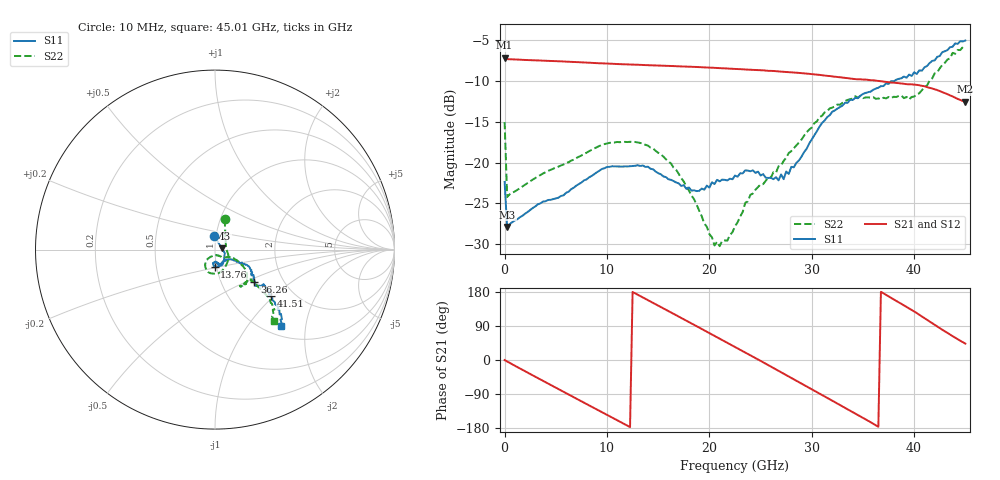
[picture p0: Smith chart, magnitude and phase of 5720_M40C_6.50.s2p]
! Device:  ADRF5720
! Description: 0.5dB LSB GaAs MMIC 6-bit Digital Attenuator
! Frequency:  0.000009 -  40 GHz
! Ports:
!	RF1	= Port 1
!	RF2	= Port 2
! Vdd:  3.3 Volt
! Vss:  -3.3 Volt
! Control:  0/3.3 Volt
! State:  6.50 dB attenuation
! Data:  The device was measured using G-S-G Probes on a matrix board.
!  Data was collected using an calibrated 4 port network analyzer.
!  The reference plane for this measurement is at the launchers.
! Note:  Analog Devices supplies this data as a sample of measured data
!  for this product.  Your particular data for this product may vary.
!  Data was taken at -40 degrees C.
!  Analog Devices reserves the right to change this data at anytime.
# GHZ S DB R 45.0
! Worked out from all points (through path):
!   181 points, 10 MHz to 45.01 GHz, reference 45 ohm
!   highest |S21| = -7.14 dB at 10 MHz (marker M1); lowest = -12.5 dB at 45.01 GHz (marker M2)
!   group delay of S21, straight-line fit = 41.3 ps
!   lowest |S11| = -27.9 dB at 260 MHz (marker M3), VSWR 1.08, Z = 48.7 + j0.608 ohm
!   |S11| at or under -10 dB: start of sweep to 38.04 GHz
!   |S22| runs from -30.2 to -5.8 dB; largest |S21 - S12| = 0.0017
!   S11 on the Smith chart (normalised r, x): 10 MHz: 0.98, +0.15; 13.76 GHz: 0.98, -0.19; 36.26 GHz: 1.43, -0.56; 41.51 GHz: 1.55, -0.97; 45.01 GHz: 1.18, -1.46
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0.01  -22.36 93.8  -7.14 -0.2  -7.16 -0.2  -15.03 72.3
0.26  -27.89 8.9  -7.31 -4.0  -7.32 -4.0  -24.20 4.5
2.26  -26.04 -11.8  -7.42 -33.3  -7.44 -33.4  -22.49 -16.7
4.26  -24.57 -21.9  -7.52 -62.3  -7.54 -62.3  -21.00 -31.5
6.01  -23.69 -36.6  -7.61 -87.5  -7.63 -87.5  -20.05 -46.2
7.76  -22.17 -49.7  -7.71 -112.6  -7.73 -112.6  -18.93 -61.3
11.01  -20.46 -71.5  -7.91 -159.1  -7.92 -159.1  -17.46 -87.0
13.76  -20.52 -91.2  -8.04 161.6  -8.06 161.5  -17.81 -108.4
15.26  -21.41 -96.2  -8.10 139.9  -8.12 139.8  -18.99 -118.6
17.76  -23.21 -92.4  -8.22 103.8  -8.25 103.7  -22.93 -127.5
20.51  -22.62 -80.6  -8.38 63.7  -8.40 63.6  -30.14 -91.9
21.76  -22.18 -75.9  -8.46 45.4  -8.48 45.3  -29.55 -67.5
22.76  -21.72 -77.2  -8.52 30.8  -8.55 30.7  -27.31 -53.7
24.01  -21.05 -70.8  -8.61 12.5  -8.63 12.4  -23.94 -44.6
27.26  -22.02 -46.2  -8.86 -35.8  -8.88 -36.0  -19.79 -25.0
30.26  -16.64 -26.9  -9.17 -81.1  -9.20 -81.2  -15.16 -30.4
33.01  -13.00 -28.9  -9.57 -122.5  -9.60 -122.7  -12.66 -40.1
36.26  -10.92 -39.6  -9.94 -172.2  -9.97 -172.3  -12.17 -53.9
37.76  -10.00 -40.5  -10.18 164.3  -10.20 164.1  -12.09 -54.4
39.51  -9.20 -36.3  -10.39 136.5  -10.41 136.3  -12.25 -43.2
41.51  -7.80 -39.6  -10.83 101.6  -10.85 101.4  -9.96 -40.7
45.01  -5.02 -49.3  -12.53 43.1  -12.56 43.0  -5.77 -50.6
